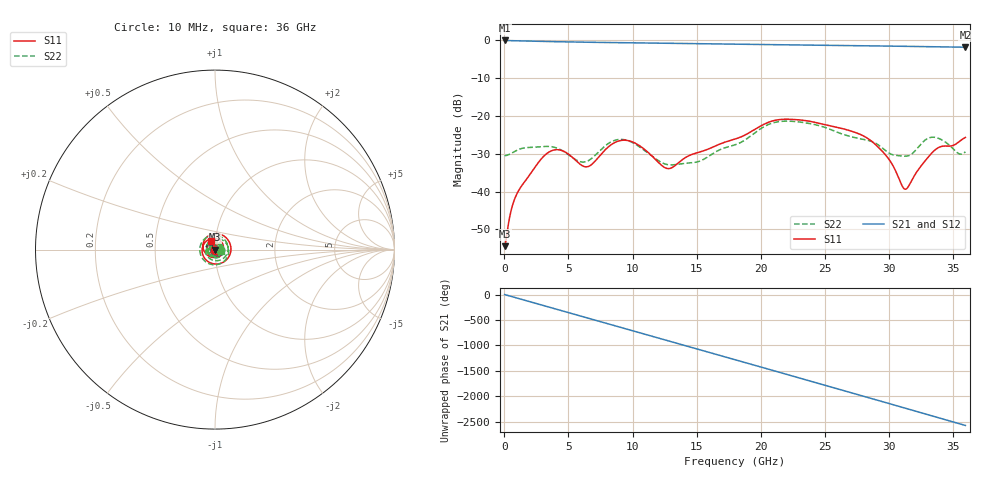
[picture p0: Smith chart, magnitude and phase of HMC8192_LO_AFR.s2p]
! Analog Devices, Inc.
! 1 Analog Way
! Wilmington, MA 01887
! http://www.analog.com
! Date:  2021-09-17 NN
! Board Name:  EVALHMC8192LG Revision A with HMC8192LG installed
! File Description:  Automatic Fixture Removal S-Parameters for LO Port connector and board loss de-embedding
! File Generation:  Calibrated Network Analyzer
! Chip Part Number:  HMC8192
! Chip Description:  Wideband IQ Mixer
! Chip Frequency:  20 to 42 GHz
! Chip Package:  LGA_CAV, 4 x 4 x 1.55 mm
! LO Port:  HMC8192LG removed and end of trace left open
! Note:
!  Analog Devices supplies this data as a sample of measured data at the evaluation board
!  ports for this product.  Your particular data for this product may vary.
!  Analog Devices reserves the right to change this data at anytime.
!  All lines below in this file are as is from the Network Analyzer.
!Agilent Technologies,N5245A,MY52451809,A.10.47.06
!Automatic Fixture Removal (AFR)
!Date: Friday, September 17, 2021 3:03:08 AM
!S2P File: Measurements: S11,S21,S12,S22:
# MHz S  RI  R 50
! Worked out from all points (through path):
!   3600 points, 10 MHz to 36 GHz, reference 50 ohm
!   highest |S21| = 0.00 dB at 10 MHz (marker M1); lowest = -1.8 dB at 36 GHz (marker M2)
!   group delay of S21, straight-line fit = 199 ps
!   lowest |S11| = -54.5 dB at 10 MHz (marker M3), VSWR 1.00, Z = 49.8 + j0.0119 ohm
!   |S11| at or under -10 dB: start of sweep to end of sweep
!   |S22| runs from -33.0 to -21.4 dB; largest |S21 - S12| = 1.5e-15
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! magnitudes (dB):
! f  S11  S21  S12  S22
! 10 MHz  -54.5  0.0  0.0  -30.5
! 520 MHz  -45.0  -0.1  -0.1  -29.9
! 910 MHz  -41.0  -0.1  -0.1  -29.2
! 3.03 GHz  -30.8  -0.3  -0.3  -28.1
! 4.34 GHz  -29.0  -0.3  -0.3  -28.9
! 6.01 GHz  -33.0  -0.4  -0.4  -32.2
! 6.68 GHz  -33.1  -0.5  -0.5  -31.5
! 8.21 GHz  -27.9  -0.6  -0.6  -27.1
! 9.29 GHz  -26.4  -0.6  -0.6  -26.2
! 10.47 GHz  -27.7  -0.6  -0.6  -28.0
! 12.01 GHz  -32.2  -0.7  -0.7  -31.8
! 12.96 GHz  -33.8  -0.8  -0.8  -33.0
! 15.15 GHz  -29.6  -0.9  -0.9  -32.1
! 18.01 GHz  -26.1  -1.0  -1.0  -27.6
! 21.03 GHz  -21.2  -1.1  -1.1  -21.8
! 24.01 GHz  -21.5  -1.2  -1.2  -22.1
! 27.94 GHz  -25.1  -1.4  -1.4  -26.1
! 30.01 GHz  -31.4  -1.5  -1.5  -29.8
! 31.35 GHz  -39.4  -1.6  -1.6  -30.6
! 33.42 GHz  -29.6  -1.7  -1.7  -25.6
! 35.48 GHz  -26.9  -1.8  -1.8  -30.0
! 36 GHz  -25.7  -1.8  -1.8  -29.5
